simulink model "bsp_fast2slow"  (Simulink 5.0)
settings: Solver=FixedStepDiscrete  StartTime=0.0  StopTime=20.0  RelTol=1e-3
libraries: simulink x1

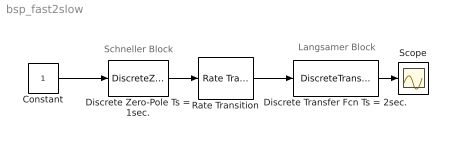
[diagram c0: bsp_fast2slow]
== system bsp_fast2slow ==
  note: Langsamer Block
  note: Schneller Block
  Constant : Constant
  Discrete Transfer Fcn Ts = 2sec. : DiscreteTransferFcn  Denominator=[1 0.5 1]  SampleTime=2
  Discrete Zero-Pole Ts = 1sec. : DiscreteZeroPole  Poles=[0 0 0.1]  Gain=2
  Rate Transition : simulink/Signal Attributes/Rate Transition  DataIntegrity=on  DeterministicTransfer=on  TransitionType=Fast to slow  InitCond=0
  Scope : Scope
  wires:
  Discrete Transfer Fcn Ts = 2sec./1 -> Scope/1
  Constant/1 -> Discrete Zero-Pole Ts = 1sec./1
  Rate Transition/1 -> Discrete Transfer Fcn Ts = 2sec./1
  Discrete Zero-Pole Ts = 1sec./1 -> Rate Transition/1
